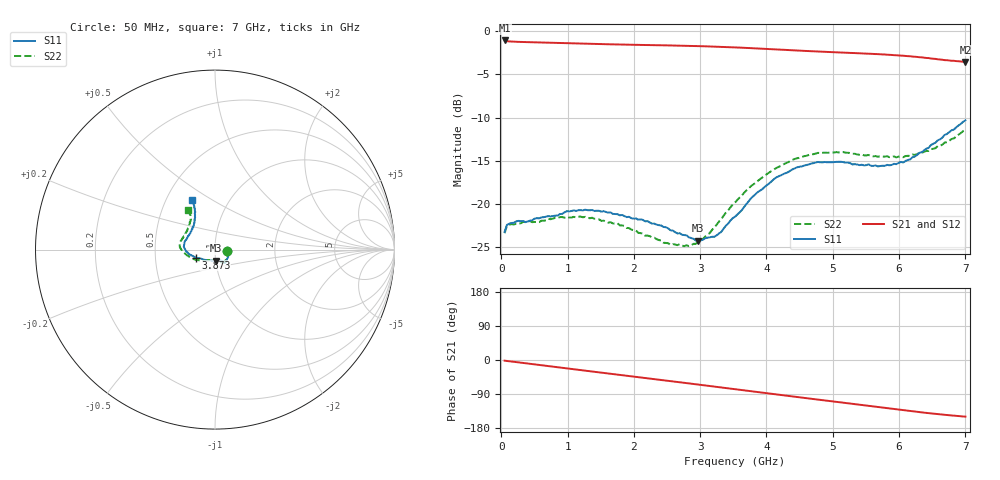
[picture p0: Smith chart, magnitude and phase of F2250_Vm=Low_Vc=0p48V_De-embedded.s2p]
! Integrated Device Technology
! Corporate Headquarters
! 6024 Silver Creek Valley Road
! San Jose, CA 95138  USA
! Phone:  1-408-284-8200
! Toll Free:  1-800-223-1366
! Webpage:  http://www.idt.com/
! Timing and RF Division
! 515 Groton Road, Suite 102
! Westford, MA 01886-6024
! Device:  F2250
! Description: Voltage Variable RF Attenuator
! Frequency:  50.0 -  6000.00 MHz
! Package:  3x3 mm Thin QFN Plastic Package: 16 pin
! Ports:  2 RF, 3 DC
!  Pin  1  = GND
!  Pin  2  = NC
!  Pin  3  = RF1  = Port 1
!  Pin  4  = NC
!  Pin  5  = GND
!  Pin  6  = GND
!  Pin  7  = GND
!  Pin  8  = GND
!  Pin  9  = NC
!  Pin 10  = RF2  = Port 2
!  Pin 11  = NC
!  Pin 12  = GND
!  Pin 13  = GND
!  Pin 14  = VCNTRL
!  Pin 15  = VDD
!  Pin 16  = VMODE
! Vcntrl:  0.480 Volts
! Vmode:  +0.000 Volts
! Vdd:  +3.30  Volts
! Current:  1.127 mA
! Data:  The device was measured on a the F2250 evaluation board which has
!  individual transmission lines to the RF pins.  Data was collected
!  using a calibrated network analyzer.  The evaluation board was
!  de-embedded using a TRL calibration technique.
!  The reference plane is the edge of the package pin.
! Misc:  SN 10
!  Action Tracker AT0258
! Date Measured:  2014-11-26
! Date:  2015-10-15  MJV
! Note:
!  Integrated Device Technology supplies this data as a sample of measured
!  data at the package pin for this product.  Your particular data for this
!  product may vary.
!  Data was taken at 25 degrees C.
!  Integrated Device Technology reserves the right to change this data at anytime.
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# GHz S dB R 50
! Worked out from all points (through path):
!   201 points, 50 MHz to 7 GHz, reference 50 ohm
!   highest |S21| = -1.06 dB at 50 MHz (marker M1); lowest = -3.5 dB at 7 GHz (marker M2)
!   group delay of S21, straight-line fit = 60.1 ps
!   lowest |S11| = -24.3 dB at 2.969 GHz (marker M3), VSWR 1.13, Z = 50.1 - j6.14 ohm
!   |S11| at or under -10 dB: start of sweep to end of sweep
!   |S22| runs from -24.9 to -11.4 dB; largest |S21 - S12| = 0.00041
!   S11 on the Smith chart (normalised r, x): 50 MHz: 1.15, -0.02; 3.873 GHz: 0.80, -0.07; 7 GHz: 0.67, +0.41
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0.05  -23.24 -8.0  -1.06 -1.8  -1.06 -1.8  -23.42 -8.8
0.08475  -22.45 -8.0  -1.14 -2.5  -1.13 -2.5  -22.57 -8.2
0.15425  -22.22 -10.1  -1.18 -4.0  -1.18 -4.0  -22.35 -10.0
0.6755  -21.50 -31.8  -1.31 -15.4  -1.31 -15.4  -21.91 -33.9
0.884  -21.19 -40.6  -1.35 -20.0  -1.35 -20.0  -21.54 -43.8
1.2315  -20.77 -50.4  -1.43 -27.4  -1.43 -27.4  -21.57 -56.4
1.75275  -21.21 -57.1  -1.52 -38.5  -1.52 -38.5  -22.26 -64.8
2.37825  -22.48 -58.7  -1.61 -51.8  -1.61 -51.8  -24.21 -70.1
2.7605  -23.63 -71.2  -1.67 -60.2  -1.67 -60.2  -24.92 -87.4
2.969  -24.26 -85.7  -1.71 -64.8  -1.71 -64.8  -24.43 -103.4
3.247  -23.66 -113.5  -1.78 -71.0  -1.77 -71.0  -22.43 -126.4
3.525  -21.51 -138.7  -1.86 -77.2  -1.86 -77.2  -19.85 -143.5
3.8725  -18.62 -157.6  -1.99 -84.8  -1.99 -84.8  -17.32 -159.3
4.1505  -16.93 -168.6  -2.10 -90.9  -2.10 -90.9  -15.84 -169.6
4.4285  -15.89 -176.7  -2.21 -96.9  -2.21 -96.9  -14.79 -177.0
4.7065  -15.29 176.3  -2.31 -103.0  -2.31 -103.0  -14.25 176.8
5.15825  -15.17 165.4  -2.47 -112.7  -2.47 -112.7  -14.01 167.4
5.85325  -15.54 141.9  -2.72 -127.6  -2.72 -127.6  -14.59 152.0
6.166  -14.86 130.5  -2.89 -134.4  -2.89 -134.5  -14.44 143.0
6.444  -13.52 121.6  -3.10 -140.2  -3.10 -140.3  -13.87 133.6
6.82625  -11.39 115.4  -3.42 -146.9  -3.42 -146.9  -12.42 125.5
7  -10.33 114.6  -3.54 -149.5  -3.54 -149.6  -11.41 124.0
